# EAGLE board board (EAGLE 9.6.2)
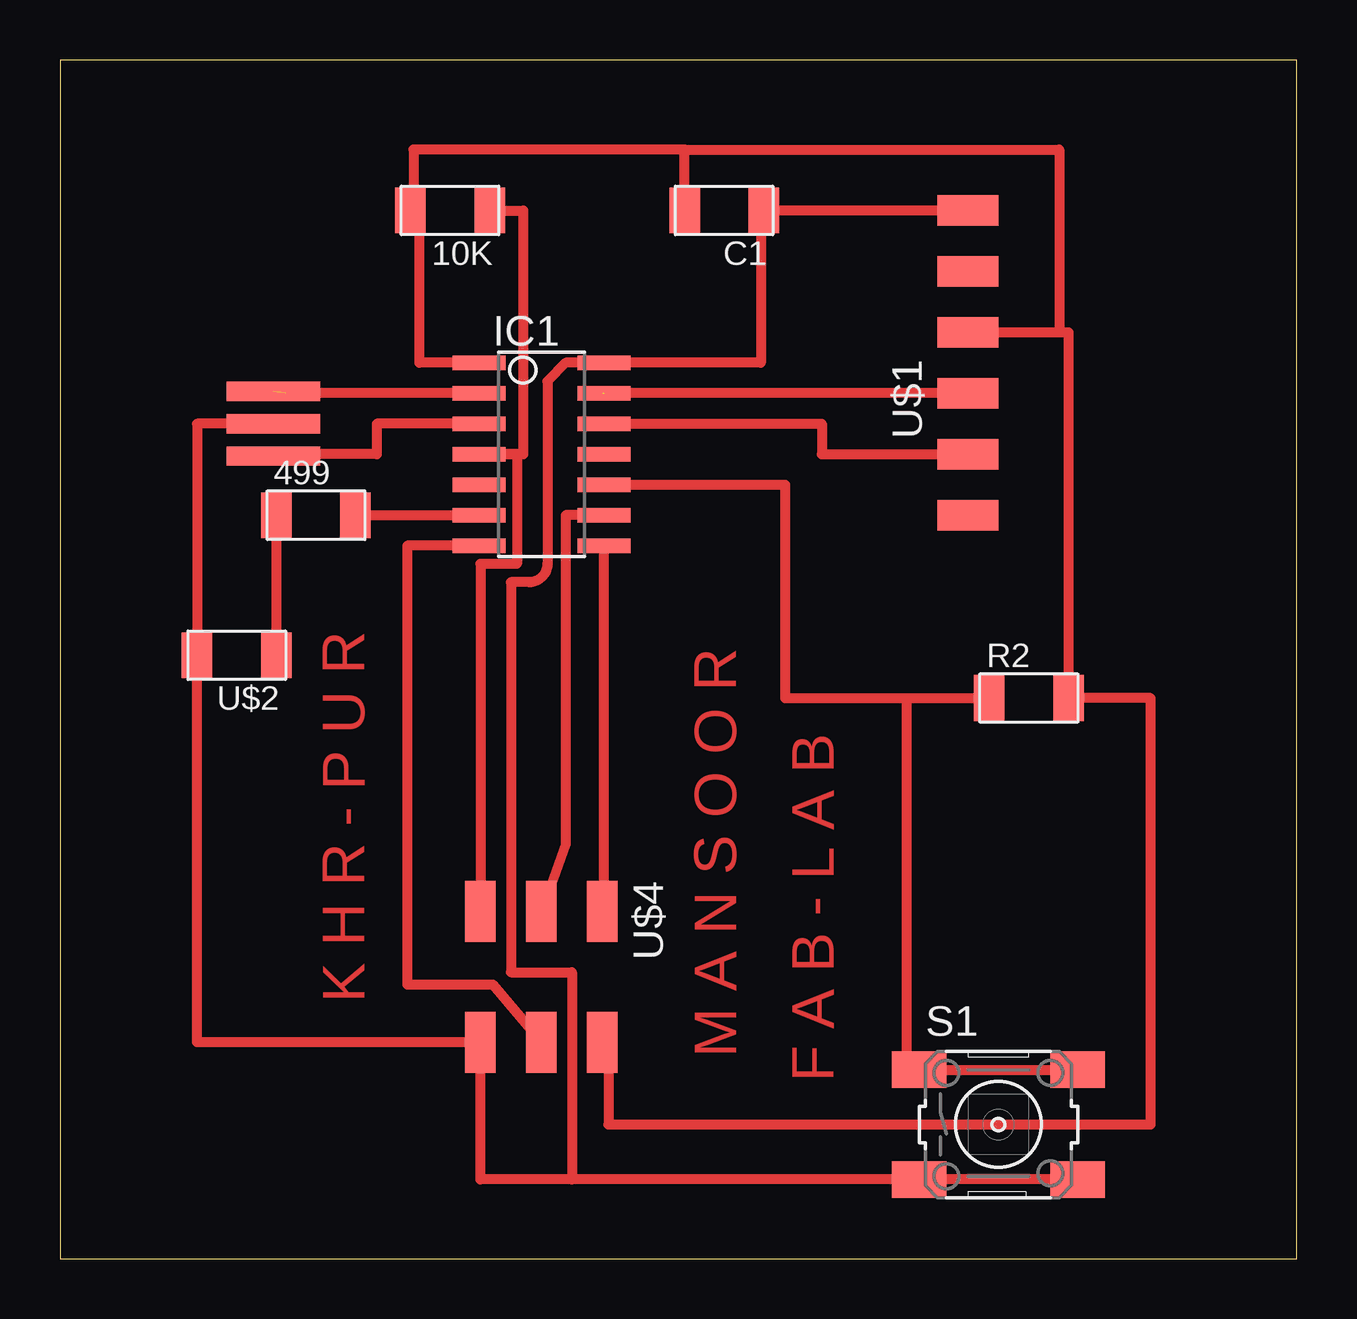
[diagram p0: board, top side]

Size 51.54 x 49.96 mm. Coordinates in mm from the lower left corner, seen from the top.
Outline: 0,0 51.54,0 51.54,49.96 0,49.96 0,0
Copper layers (1*16): Top 0.035mm / dielectric 1.5mm / Bottom 0.035mm
Design rules "default": minimum track width 10mil, minimum drill 24mil, track to track 8mil, track to pad 8mil, pad to pad 8mil, via to via 8mil, smd to smd 8mil, copper to edge 40mil, drill to drill 8mil, minimum pad ring 10mil, minimum via ring 8mil, stop-mask expansion 4mil, vias tented up to drill 0mil, thermal gap 10mil

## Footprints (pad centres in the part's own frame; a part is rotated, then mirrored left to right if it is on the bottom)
R1206FAB = smd 1.27 x 1.905: 1 -1.651,0; 2 1.651,0
C1206FAB = smd 1.27 x 1.905: 1 -1.651,0; 2 1.651,0
SOIC14 = smd 0.61 x 2.21: 1 -3.81,-2.603; 2 -2.54,-2.603; 3 -1.27,-2.603; 4 0,-2.603; 5 1.27,-2.603; 6 2.54,-2.603; 7 3.81,-2.603; 8 3.81,2.603; 9 2.54,2.603; 10 1.27,2.603; 11 0,2.603; 12 -1.27,2.603; 13 -2.54,2.603; 14 -3.81,2.603
6MM_SWITCH = smd 2.286 x 1.524: 1 -3.302,2.286; 2 3.302,2.286; 3 -3.302,-2.286; 4 3.302,-2.286
1X06SMD = smd 2.54 x 1.27: 1 0,6.35; 2 0,3.81; 3 0,1.27; 4 0,-1.27; 5 0,-3.81; 6 0,-6.35
LED1206FAB = smd 1.27 x 1.905: 1 -1.651,0; 2 1.651,0
EFOBM = smd 0.8 x 3.9: 1 -1.35,0; 2 0,0; 3 1.35,0
2X03SMD = smd 2.54 x 1.27: 1 -2.54,2.54; 2 2.92,2.54; 3 -2.54,0; 4 2.92,0; 5 -2.54,-2.54; 6 2.92,-2.54

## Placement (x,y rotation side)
10K  R  [R1206FAB]  16.26,43.69 180 top
499  [R1206FAB]  10.67,30.99 0 top
C1  [C1206FAB]  27.69,43.69 180 top
IC1  ATTINY44-SSU  [SOIC14]  20.07,33.53 270 top
R2  10k  [R1206FAB]  40.39,23.37 0 top
S1  [6MM_SWITCH]  39.12,5.59 0 top
U$1  FTDI-SMD-HEADER  [1X06SMD]  37.85,37.34 0 top
U$2  LEDFAB1206  [LED1206FAB]  7.37,25.15 180 top
U$3  RESONATOR  [EFOBM]  8.89,34.8 270 top
U$4  AVRISPSMD  [2X03SMD]  20.07,11.94 270 top

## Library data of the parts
10K 499 C1 IC1 R2 S1 U$1-U$4 = fab

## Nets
BUTTON: IC1.10 R2.1 S1.1 S1.2
CTS: U$1.2
GND: C1.1 IC1.14 S1.3 S1.4 U$1.1 U$2.2 U$3.2 U$4.6
LED: 499.2 IC1.6
MISO: IC1.8 U$4.1
MOSI: IC1.7 U$4.4
N$4: IC1.2 U$3.1
N$5: IC1.3 U$3.3
N$6: 499.1 U$2.1
RST: 10K.1 IC1.4 U$4.5
RTS: U$1.6
RXD: IC1.12 U$1.5
SCK: IC1.9 U$4.3
TXD: IC1.13 U$1.4
VCC: 10K.2 C1.2 IC1.1 R2.2 U$1.3 U$4.2

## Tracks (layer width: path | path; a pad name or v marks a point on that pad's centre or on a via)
BUTTON
  Top 0.406: IC1.10 30.23,32.26 30.23,23.37 35.31,23.37 | 35.31,23.37 R2.1 | 35.31,23.37 35.31,7.87 S1.1 S1.2
GND
  Top 0.406: U$1.1 C1.1 29.21,43.69 29.21,37.34 IC1.14 21.08,37.34 20.32,36.58 20.32,28.96 arc-90 19.56,28.19 18.8,28.19 18.8,11.94 21.34,11.94 21.34,3.3 | U$3.2 5.71,34.8 U$2.2 5.71,9.02 U$4.6 17.53,3.3 21.34,3.3 | 21.34,3.3 S1.3 S1.4
LED
  Top 0.406: 499.2 IC1.6
MISO
  Top 0.406: U$4.1 22.67,14.48 IC1.8
MOSI
  Top 0.406: IC1.7 14.48,29.72 14.48,11.43 18.03,11.43 U$4.4
N$4  (1 unrouted)
  Top 0.406: IC1.2 9.4,36.07
N$5
  Top 0.406: IC1.3 13.21,34.8 13.21,33.53 8.89,33.53 U$3.3
N$6
  Top 0.406: 499.1 U$2.1
RST
  Top 0.406: 10K.1 19.3,43.69 19.3,33.53 IC1.4 19.05,33.53 19.05,28.96 17.53,28.96 U$4.5
RXD
  Top 0.406: IC1.12 31.75,34.8 31.75,33.53 U$1.5
SCK
  Top 0.406: IC1.9 21.08,30.99 21.08,17.27 U$4.3
TXD  (1 unrouted)
  Top 0.406: U$1.4 22.61,36.07
VCC
  Top 0.406: U$1.3 41.66,38.61 | 26.03,46.23 41.66,46.23 41.66,38.61 | 41.66,38.61 42.04,38.61 R2.2 45.47,23.37 45.47,5.59 27.94,5.59 27.31,5.59 22.86,5.59 22.86,9.02 U$4.2 | C1.2 26.03,46.23 | 26.03,46.23 14.73,46.23 14.73,43.69 10K.2 14.6,43.18 14.99,43.18 14.99,37.34 IC1.1

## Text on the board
Top: K H R - P U R | M A N S O O R | F A B - L A B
